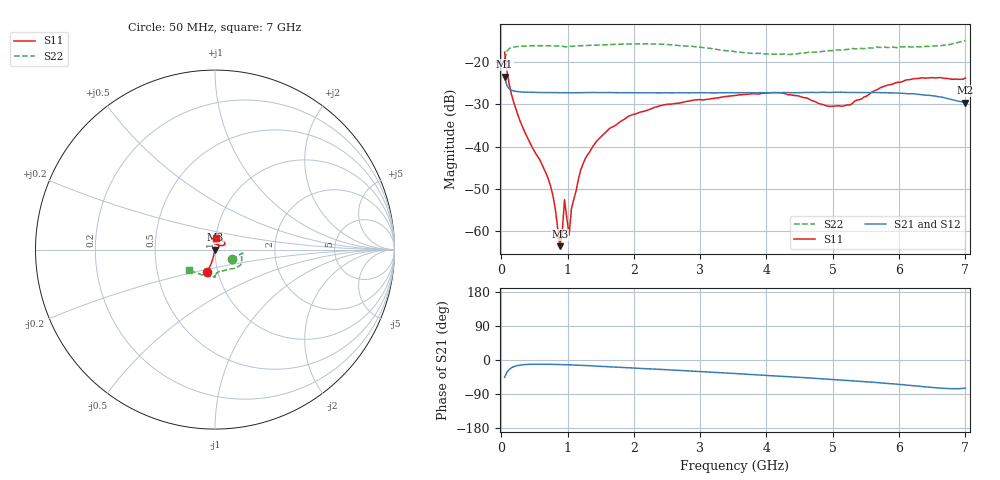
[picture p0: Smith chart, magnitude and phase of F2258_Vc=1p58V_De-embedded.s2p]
! Integrated Device Technology
! Corporate Headquarters
! 6024 Silver Creek Valley Road
! San Jose, CA 95138  USA
! Phone:  1-408-284-8200
! Toll Free:  1-800-223-1366
! Webpage:  http://www.idt.com/
! Timing and RF Division
! 515 Groton Road, Suite 102
! Westford, MA 01886-6024
! Device:  F2258
! Description: Voltage Variable RF Attenuator
! Frequency:  50.0 -  6000.00 MHz
! Package:  3x3 mm Thin QFN Plastic Package: 16 pin
! Ports:  2 RF, 2 DC
!  Pin  1  = NC
!  Pin  2  = NC
!  Pin  3  = RF2  = Port 2
!  Pin  4  = GND
!  Pin  5  = Vdd
!  Pin  6  = NC
!  Pin  7  = VCTRL
!  Pin  8  = NC
!  Pin  9  = GND
!  Pin 10  = RF1  = Port 1
!  Pin 11  = NC
!  Pin 12  = NC
!  Pin 13  = NC
!  Pin 14  = NC
!  Pin 15  = NC
!  Pin 16  = NC
! Vcntrl:  1.580 Volts
! Vdd:  +3.300 Volts
! Current:  1.161 mA
! Data:  The device was measured on a the F2258 evaluation board which has
!  individual transmission lines to the RF pins.  Data was collected
!  using a calibrated network analyzer.  The evaluation board was
!  de-embedded using a TRL calibration technique.
!  The reference plane is the edge of the package pin.
! Misc:  SN 10
!  Action Tracker AT0285
! Date Measured:  2014-12-10
! Date:  2016-01-13  MJV
! Note:
!  Integrated Device Technology supplies this data as a sample of measured
!  data at the package pin for this product.  Your particular data for this
!  product may vary.
!  Data was taken at 25 degrees C.
!  Integrated Device Technology reserves the right to change this data at anytime.
!Freq_(GHz)  S11M_(dB)  S11P_(deg)  S21M_(dB)  S21P_(deg)  S12M_(dB)  S12P_(deg)  S22M_(dB)  S22P_(deg)
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# GHz S dB R 50
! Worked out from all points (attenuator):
!   201 points, 50 MHz to 7 GHz, reference 50 ohm
!   highest |S21| = -23.37 dB at 50 MHz (marker M1); lowest = -29.5 dB at 7 GHz (marker M2)
!   lowest |S11| = -63.6 dB at 884 MHz (marker M3), VSWR 1.00, Z = 50.1 - j0.0225 ohm
!   |S11| at or under -10 dB: start of sweep to end of sweep
!   |S22| runs from -19.3 to -14.8 dB; largest |S21 - S12| = 0.00023
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0.05  -17.56 -109.2  -23.37 -45.8  -23.38 -45.8  -19.28 -30.0
0.1195  -25.18 -103.4  -26.27 -24.8  -26.27 -24.8  -16.75 -9.9
0.2585  -32.84 -104.1  -26.97 -14.2  -26.97 -14.2  -16.24 -7.1
0.745  -49.45 -98.4  -27.19 -11.4  -27.19 -11.4  -16.12 -12.1
0.8145  -54.74 -85.0  -27.18 -11.7  -27.20 -11.7  -16.11 -13.1
0.884  -63.58 -19.9  -27.22 -12.0  -27.20 -12.0  -16.15 -14.5
0.91875  -60.27 23.8  -27.21 -12.2  -27.20 -12.2  -16.15 -15.0
0.9535  -52.57 -114.2  -27.20 -12.4  -27.20 -12.4  -16.33 -14.8
1.023  -60.94 -48.4  -27.24 -12.8  -27.22 -12.8  -16.25 -16.2
1.05775  -54.73 -12.7  -27.23 -13.0  -27.19 -13.0  -16.22 -16.6
1.2315  -44.15 18.7  -27.17 -14.2  -27.15 -14.3  -16.05 -19.1
1.44  -38.63 20.1  -27.18 -16.2  -27.21 -16.2  -15.93 -21.9
1.6485  -35.53 23.5  -27.17 -18.1  -27.19 -18.1  -15.79 -24.7
2.37825  -30.36 42.3  -27.25 -24.6  -27.27 -24.6  -15.69 -33.9
3.525  -27.90 88.9  -27.22 -35.7  -27.19 -35.8  -17.48 -56.3
4.1505  -27.17 103.8  -27.18 -42.2  -27.18 -42.2  -18.02 -74.5
4.7065  -29.16 94.2  -27.12 -48.1  -27.11 -48.1  -17.64 -85.3
4.94975  -30.45 77.6  -27.15 -50.7  -27.13 -50.7  -17.25 -87.6
5.2625  -30.13 50.2  -27.16 -54.4  -27.15 -54.4  -16.84 -89.3
5.85325  -25.34 27.2  -27.25 -62.3  -27.26 -62.3  -16.49 -91.1
6.33975  -23.67 33.0  -27.69 -70.0  -27.67 -70.0  -16.35 -101.6
7  -23.73 83.5  -29.54 -74.4  -29.54 -74.3  -14.82 -142.1
